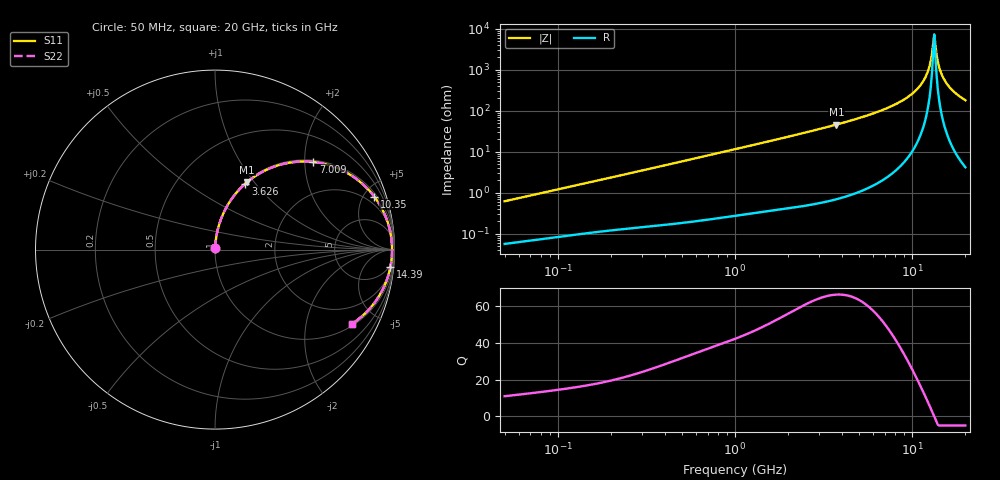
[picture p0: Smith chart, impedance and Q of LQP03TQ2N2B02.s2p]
!Murata Part Number: LQP03TQ2N2B02
!These Parameters are Measured in Series Mode Connection
!  o--[Z]--o
!Port1  Port2
!  o-------o
!Freq. Start=50[MHz] Stop=20[GHz], 401[Steps]
# Hz S RI R 50
!Freq.(Hz) S11(Real) S11(Imag) S21(Real) S21(Imag) S12(Real) S12(Imag) S22(Real) S22(Imag)
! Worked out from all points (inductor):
!   401 points, 50 MHz to 20 GHz, reference 50 ohm
!   read as one part in series: L = 1.96 nH near 51.52 MHz
!   highest Q = 66.3 at 3.736 GHz (marker M1), where L = 1.97 nH
!   self-resonance near 13.15 GHz
!   S11 on the Smith chart (normalised r, x): 50 MHz: 1.00, +0.01; 3.626 GHz: 1.01, +0.89; 7.009 GHz: 1.04, +2.21; 10.35 GHz: 1.26, +5.91; 14.39 GHz: 4, -20; 20 GHz: 1.08, -3.64
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5e7  0.000605 0.0062  0.9994 -0.0062  0.9994 -0.0062  0.000605 0.0062
1.364002e8  0.00126 0.0163  0.9987 -0.0163  0.9987 -0.0163  0.00126 0.0163
3.721004e8  0.00347 0.0432  0.9965 -0.0432  0.9965 -0.0432  0.00347 0.0432
1e9  0.0159 0.1137  0.9841 -0.1137  0.9841 -0.1137  0.0159 0.1137
2.728004e9  0.0993 0.2912  0.9007 -0.2912  0.9007 -0.2912  0.0993 0.2912
3.626126e9  0.1699 0.368  0.8301 -0.368  0.8301 -0.368  0.1699 0.368
3.736399e9  0.1797 0.3765  0.8203 -0.3765  0.8203 -0.3765  0.1797 0.3765
5.194772e9  0.3299 0.4622  0.6701 -0.4622  0.6701 -0.4622  0.3299 0.4622
7.009217e9  0.5478 0.4879  0.4522 -0.4879  0.4522 -0.4879  0.5478 0.4879
7.442007e9  0.6002 0.4793  0.3998 -0.4793  0.3998 -0.4793  0.6002 0.4793
8.907419e9  0.7639 0.4105  0.2361 -0.4105  0.2361 -0.4105  0.7639 0.4105
1.034674e10  0.8873 0.2952  0.1127 -0.2952  0.1127 -0.2952  0.8873 0.2952
1.131968e10  0.9429 0.2013  0.0571 -0.2013  0.0571 -0.2013  0.9429 0.2013
1.201863e10  0.9685 0.1307  0.0315 -0.1307  0.0315 -0.1307  0.9685 0.1307
1.257102e10  0.9806 0.0749  0.0194 -0.0749  0.0194 -0.0749  0.9806 0.0749
1.295331e10  0.9851 0.0368  0.0149 -0.0368  0.0149 -0.0368  0.9851 0.0368
1.334722e10  0.9866 -0.00158  0.0134 0.00158  0.0134 0.00158  0.9866 -0.00158
1.375312e10  0.985 -0.04  0.015 0.04  0.015 0.04  0.985 -0.04
1.438523e10  0.9772 -0.0969  0.0228 0.0969  0.0228 0.0969  0.9772 -0.0969
1.504638e10  0.9629 -0.152  0.0371 0.152  0.0371 0.152  0.9629 -0.152
1.621653e10  0.9261 -0.2377  0.0739 0.2377  0.0739 0.2377  0.9261 -0.2377
2e10  0.7628 -0.414  0.2372 0.414  0.2372 0.414  0.7628 -0.414
